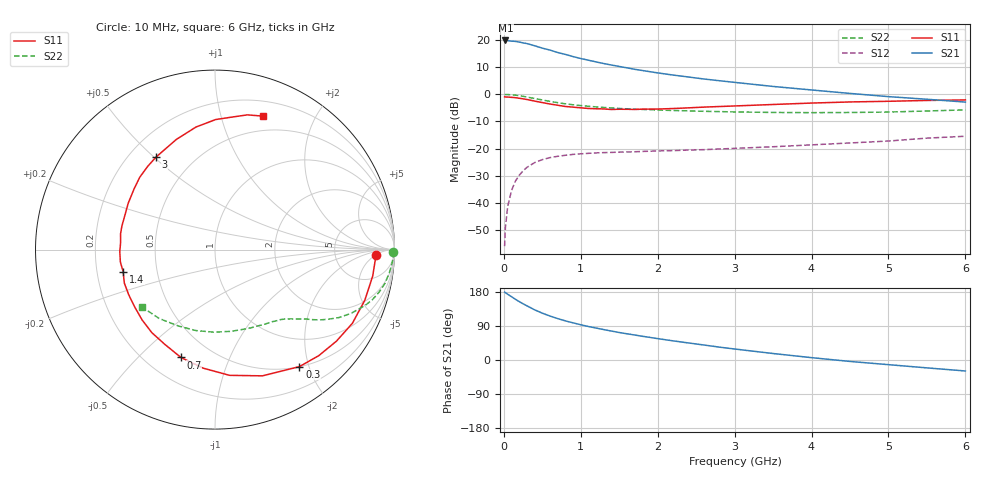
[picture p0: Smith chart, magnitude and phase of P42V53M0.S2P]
! SIEMENS Small Signal Semiconductors
! BFP182
! Si NPN RF Bipolar Junction Transistor in SOT143
! VCE = 2.5 V  IC = 3 mA
! Common Emitter S-Parameters:  March  1996
# GHz  S  MA  R  50
!  f  S11  S21  S12  S22
! GHz  MAG  ANG  MAG  ANG  MAG  ANG  MAG  ANG
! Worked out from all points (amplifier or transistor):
!   36 points, 10 MHz to 6 GHz, reference 50 ohm
!   highest |S21| = 19.8 dB at 20 MHz (marker M1)
!   |S21| within 3 dB of that: start of sweep to 524.4 MHz
!   unconditionally stable (mu >= 1): 1.913 GHz to 5.709 GHz
!   at 250 MHz: K = 0.16, MSG = 23.6 dB, |S12| = -28.2 dB
!   at 1.4 GHz: K = 0.79, MSG = 16.1 dB, |S12| = -21.4 dB
!   at 6 GHz: K = 0.97, MSG = 6.3 dB, |S12| = -15.4 dB
!   S11 on the Smith chart (normalised r, x): 10 MHz: 17, -5; 300 MHz: 0.50, -1.85; 700 MHz: 0.34, -0.68; 1.4 GHz: 0.31, -0.11; 3 GHz: 0.31, +0.51; 6 GHz: 0.34, +1.36
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0.01  0.8969 -1.9  9.688 179.0  0.0016 91.2  0.9933 -0.7
0.02  0.8946 -3.8  9.827 177.9  0.0035 89.7  0.9922 -1.5
0.05  0.891 -9.5  9.756 173.4  0.0086 86.3  0.9914 -3.8
0.1  0.8811 -18.6  9.534 167.0  0.017 78.1  0.9798 -7.6
0.15  0.8687 -28.2  9.452 160.3  0.0252 74.2  0.9656 -11.2
0.2  0.8474 -37.0  9.191 154.1  0.0323 69.6  0.9447 -14.5
0.3  0.8039 -54.2  8.61 143.0  0.0452 60.6  0.8926 -20.4
0.4  0.7514 -69.4  7.846 132.4  0.0553 53.5  0.8384 -25.0
0.5  0.7052 -83.4  7.099 123.6  0.0628 47.1  0.7883 -28.7
0.6  0.6636 -95.8  6.534 116.0  0.0684 42.5  0.7419 -31.5
0.7  0.6302 -107.5  5.891 109.3  0.0723 38.5  0.7028 -33.9
0.8  0.5975 -117.9  5.437 103.2  0.0755 35.6  0.6687 -35.7
0.9  0.5814 -127.2  4.965 98.1  0.0784 32.9  0.6422 -37.1
1.1  0.5496 -144.7  4.253 88.3  0.082 28.7  0.6026 -39.9
1.4  0.5263 -166.5  3.464 76.4  0.0852 24.9  0.5614 -43.5
1.8  0.5335 170.5  2.75 62.6  0.0889 23.0  0.5275 -48.4
2.2  0.5482 151.9  2.266 50.5  0.092 22.3  0.5046 -54.3
3  0.6111 122.6  1.662 29.0  0.1011 22.3  0.4747 -68.4
3.5  0.6507 109.3  1.398 17.1  0.1084 21.9  0.464 -78.9
4.5  0.7247 89.7  1.04 -3.8  0.1273 20.8  0.4634 -103.2
5.5  0.772 76.5  0.812 -20.8  0.1562 18.3  0.4939 -129.0
6  0.79 70.3  0.72 -29.0  0.1692 14.6  0.5171 -141.7
